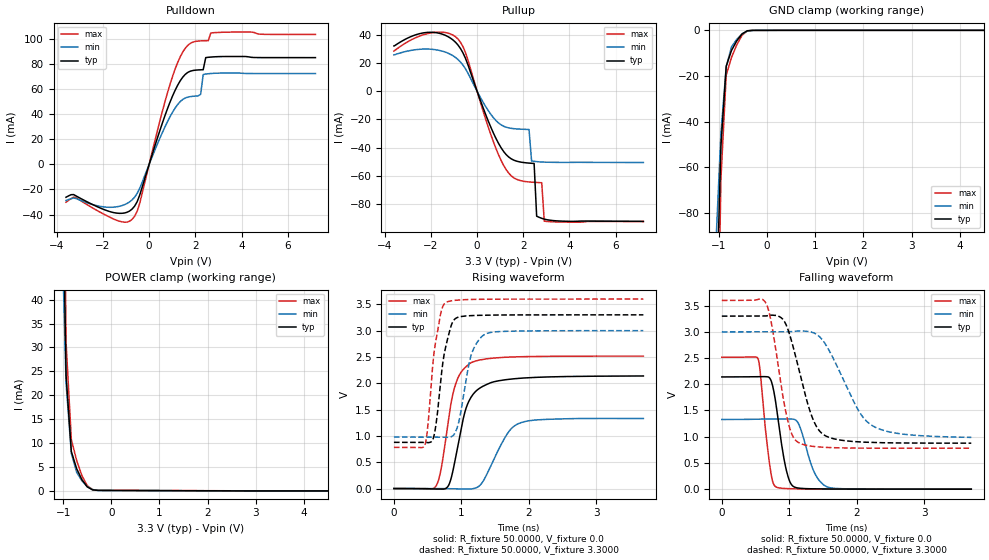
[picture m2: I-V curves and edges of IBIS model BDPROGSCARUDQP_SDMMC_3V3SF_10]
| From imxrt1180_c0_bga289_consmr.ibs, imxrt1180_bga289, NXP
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[Model]  BDPROGSCARUDQP_SDMMC_3V3SF_10
|   Model BDPROGSCARUDQP_SDMMC_3V3SF_10
| This model was characterised for following simulation conditions:
| External (pad) voltage:
|   - Typ: 3.3V,   - Min: 3.0V,   - Max: 3.6V
| Library cells for typ/min/max conditions are connected as defined below:
|  IO - External Pad
|  A - Core Input
|  EN - Output Buffer Enable
|  ASRCN3V3[0] - REFH3V3 gnde REFH3V3
|  ASRCN3V3[1] - REFH3V3 REFH3V3 gnde
|  ASRCN3V3[2] - gnde
|  ASRCN3V3[3] - gnde REFH3V3 gnde
|  ASRCP3V3[0] - vdde3v3 vdde3v3 REFL3V3
|  ASRCP3V3[1] - vdde3v3 REFL3V3 vdde3v3
|  ASRCP3V3[2] - REFL3V3 vdde3v3 vdde3v3
|  ASRCP3V3[3] - REFL3V3 REFL3V3 vdde3v3
|  IOGC - NC
|  PDRV - gnd
|  PSW - vdd
|  REFH3V3 - REFH3V3
|  REFL3V3 - REFL3V3
|  ZI - NC
|  gnd - gnd
|  gnde - gnde
|  vdd - vdd
|  vdde3v3 - vdde3v3
| All other pins connected to ground
Model_type I/O
Polarity   Non-Inverting
Enable   Active-Low
Vinl =   0.7500V
Vinh =   2.2500V
Vmeas =  1.6500V
Cref =   30.0000pF
Rref =   1.0000M
Vref =   3.3000V
C_comp   2.1236pF   2.1089pF   2.1446pF
|C_comp_pullup   0.3619pF   0.3752pF   0.3519pF
|C_comp_pulldown   0.6265pF   0.6593pF   0.5997pF
[Model Spec]
| variable   typ   min   max
Vinh   2.0625V   1.8750V   2.2500V
Vinl   0.8250V   0.7500V   0.9000V
[Temperature Range]   25.0000   0.1050k   -20.0000
[Voltage Range]   3.3000V   3.0000V   3.6000V
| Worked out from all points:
|   slope of the pulldown table from 0 to 0.495 V, typ, clamps not added: 17.2 ohm
|   slope of the pullup table from 0 to 0.495 V, typ, clamps not added: 23 ohm
|   GND clamp passes 1 mA (typ) near -0.48 V on its own axis
|   POWER clamp passes 1 mA (typ) near -0.51 V on its own axis
|   rising waveform, R_fixture 50.0000, V_fixture 0.0: 20-80 % time 243ps typ, 318ps min, 205ps max; typ from 0 V to 2.14 V
|   rising waveform, R_fixture 50.0000, V_fixture 3.3000: 20-80 % time 152ps typ, 180ps min, 140ps max; typ from 0.878 V to 3.3 V
|   falling waveform, R_fixture 50.0000, V_fixture 0.0: 20-80 % time 153ps typ, 202ps min, 120ps max; typ from 2.14 V to 0 V
|   falling waveform, R_fixture 50.0000, V_fixture 3.3000: 20-80 % time 307ps typ, 472ps min, 217ps max; typ from 3.3 V to 0.877 V
[Pulldown]
|Voltage   I(typ)   I(min)   I(max)
-3.6V     -26.23mA   -28.81mA   -30.21mA
-3.16V    -25.23mA   -27.28mA   -26.61mA
-1.4V     -38.9mA    -33.84mA   -44.66mA
-630mV    -33.34mA   -26.18mA   -41.42mA
1.02V     54.81mA    41.81mA    70.52mA
1.79V     74.36mA    54.06mA    96.61mA
2.23V     75.41mA    55.91mA    98.49mA
2.34V     75.48mA    71.67mA    98.57mA
2.45V     85.15mA    72.01mA    98.62mA
2.56V     85.39mA    72.28mA    98.66mA
2.78V     85.72mA    72.61mA    105mA
7.2V      85.14mA    72.43mA    103.6mA
[Pullup]
|Voltage   I(typ)   I(min)   I(max)
-3.6V     31.94mA    25.58mA    28.32mA
-2.04V    41.59mA    29.68mA    41.02mA
-830mV    32.67mA    22.42mA    36.89mA
-500mV    23.13mA    15.77mA    27.21mA
1.15V     -42.62mA   -24.78mA   -52.41mA
2.25V     -50.81mA   -27.06mA   -64.11mA
2.36V     -50.94mA   -49.27mA   -64.27mA
2.47V     -51.06mA   -49.56mA   -64.39mA
2.58V     -88.31mA   -49.77mA   -64.49mA
2.8V      -89.83mA   -50.03mA   -64.67mA
2.91V     -90.37mA   -50.11mA   -91.82mA
7.2V      -91.99mA   -50.37mA   -92.07mA
[GND_clamp]
|Voltage   I(typ)   I(min)   I(max)
-3.6V     -5.131A    -2.969A    -8.406A
-1.07V    -134.2mA   -96.54mA   -200.7mA
-960mV    -50.84mA   -45.29mA   -65.28mA
-850mV    -15.74mA   -15.96mA   -19.63mA
-740mV    -8.808mA   -7.274mA   -11.89mA
-630mV    -4.596mA   -3.904mA   -6.316mA
-520mV    -1.551mA   -1.569mA   -2.126mA
-410mV    -182.3uA   -313uA     -219.4uA
-190mV    -16.94uA   -13.41uA   -23.77uA
7.2V      0A         0A         0A
[POWER_clamp]
|Voltage   I(typ)   I(min)   I(max)
-3.6V     5.01A      2.85A      8.324A
-1.05V    90.64mA    63.89mA    144.9mA
-940mV    24.29mA    22.59mA    31.15mA
-830mV    8.246mA    7.833mA    10.76mA
-720mV    4.663mA    3.912mA    6.37mA
-610mV    2.344mA    2.102mA    3.186mA
-500mV    850.8uA    907.7uA    1.111mA
-390mV    222uA      289.9uA    270.2uA
-170mV    103uA      76.12uA    142.4uA
7.2V      0A         0A         0A
[Ramp]
| variable   typ   min   max
dV/dt_r  1.2825/0.2428n   0.7982/0.3178n   1.5089/0.2048n
dV/dt_f  1.4529/0.3068n   1.2068/0.4720n   1.6901/0.2167n
R_load = 50.0000
[Rising Waveform]
R_fixture= 50.0000
V_fixture= 0.0
V_fixture_min= 0.0
V_fixture_max= 0.0
|time   V(typ)   V(min)   V(max)
0s        133.3uV    116.1uV    163.4uV
629ps     -10.2mV    167.2uV    58.43mV
702.1ps   -11mV      -203.4uV   387.4mV
797.3ps   33.12mV    -2.906mV   1.196V
895ps     457mV      -7.121mV   1.898V
1.042ns   1.398V     -7.94mV    2.28V
1.143ns   1.732V     -7.678mV   2.388V
1.308ns   1.934V     111mV      2.45V
1.852ns   2.092V     1.235V     2.502V
3.7ns     2.138V     1.33V      2.515V
[Rising Waveform]
R_fixture= 50.0000
V_fixture= 3.3000
V_fixture_min= 3.0000
V_fixture_max= 3.6000
|time   V(typ)   V(min)   V(max)
0s        877.7mV    977.1mV    782.1mV
459.3ps   876.7mV    977.2mV    825.5mV
500.9ps   872.1mV    977.1mV    1.158V
599.5ps   1.03V      977.3mV    2.624V
701.9ps   2.138V     976.6mV    3.369V
776.1ps   2.736V     972.4mV    3.536V
935.8ps   3.245V     1.145V     3.578V
1.147ns   3.284V     2.538V     3.591V
1.341ns   3.292V     2.923V     3.595V
3.7ns     3.299V     2.998V     3.598V
[Falling Waveform]
R_fixture= 50.0000
V_fixture= 0.0
V_fixture_min= 0.0
V_fixture_max= 0.0
|time   V(typ)   V(min)   V(max)
0s        2.139V     1.329V     2.515V
538.9ps   2.145V     1.335V     2.479V
710.2ps   2.118V     1.337V     459.5mV
802.7ps   1.625V     1.337V     43.29mV
949.4ps   402.6mV    1.337V     11.9mV
1.084ns   36.21mV    1.326V     6.589mV
1.169ns   16mV       1.15V      4.835mV
1.37ns    6.317mV    325.6mV    2.464mV
1.556ns   3.72mV     47.04mV    1.375mV
3.7ns     140.4uV    255.3uV    164.1uV
[Falling Waveform]
R_fixture= 50.0000
V_fixture= 3.3000
V_fixture_min= 3.0000
V_fixture_max= 3.6000
|time   V(typ)   V(min)   V(max)
0s        3.299V     2.999V     3.598V
658.7ps   3.303V     2.999V     3.535V
743ps     3.317V     3V         3.115V
968.1ps   3.089V     3V         1.359V
1.134ns   2.329V     3.016V     891.4mV
1.351ns   1.336V     2.985V     815.8mV
1.561ns   1.002V     2.712V     795.3mV
2.011ns   903.2mV    1.536V     783mV
2.232ns   890.5mV    1.211V     781.6mV
3.7ns     877.1mV    987.3mV    781.4mV
